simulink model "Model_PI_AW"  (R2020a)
settings: Solver=ode15s  StartTime=0.0  StopTime=tsim  MaxStep=0.1  RelTol=1e-5
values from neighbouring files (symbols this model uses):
  C = Fc*cpc/(Fh*cph)    [calcblock.m]    (also in calcblock2.m; calcblock3.m; eNTU.m = m.c*cp.c/(m.h*cp.h); Main.m = [zeros(1,2*N-1),1])
  d_tstep = 300    [Main.m]    (also in Main_OL.m = 3000; runTestCalcBlk.m; runTransf.m = [500; 50000; 70000; 130000; 50000; 50000]; runTransfOL.m = [500 5000 7000 13000])
  dFh = 0;0.2*Fh    [Main.m]    (also in runTransf.m = 2; runTransfOL.m = 0)
  dTcin = 2    [Main.m]    (also in runTransf.m = 0; runTransfOL.m = 0)
  dThin = 0;2    [Main.m]    (also in runTransf.m = 0; runTransfOL.m = 0)
  Fc0 = 5    [Main.m]    (also in Main_OL.m; runTestCalcBlk.m; runTransf.m; runTransfOL.m)
  Fh = d(1)    [calcblock.m]    (also in calcblock2.m; calcblock3.m; HEXode.m; Main.m = 3)
  Kc = 1/k*tau/(tauC+theta)    (= -0.124875124875)    [Main.m]    (also in runTransf.m = 1/kM(i)*tau(i)/(tauCM(i)+theta(i)); runTransfOL.m = 1/kM(i)*tau(i)/(tauCM(i)+theta(i)))
  nd = size(d0,2)    [Main.m]    (also in Main_OL.m; runTestCalcBlk.m; runTransf.m = size(d0,1); runTransfOL.m)
  np = size(p,2)    [Main.m]    (also in Main_OL.m; runTestCalcBlk.m; runH2Psim.m = length(param); runTransf.m)
  nu = 1    [Main.m]    (also in Main_OL.m; runTestCalcBlk.m; runH2Psim.m = length(u0); runTransf.m)
  nx = size(x0,1)    [Main.m]    (also in Main_OL.m; runTestCalcBlk.m; H2P_Turbine_driven.m = param(end); runTD.m = length(x0))
  p = [N, Fc0, rhoc, rhoh,U,A,cpc,cph]    [Main.m]    (also in Main_OL.m; runTestCalcBlk.m; NonlinearMap.m = [U;A;Fc(i);Fh;cpc;cph;Tcin;Thin]; runTransf.m = [N, Fc0, rhoc, rhoh, U0, A,cpc,cph])
  tauI = min(tau,4*(tauC+theta))    [Main.m]    (also in runTransf.m = min(tau(i), 4*(tauCM(i)+theta(i))); runTransfOL.m = min(tau(i), 4*(tauCM(i)+theta(i))))
  Tcin = d(2)    [calcblock.m]    (also in calcblock2.m; calcblock3.m; HEXode.m; Main.m = 293.15)
  Thin = d(3)    [calcblock.m]    (also in calcblock2.m; calcblock3.m; HEXode.m; Main.m = 343.15)
  Thsp = Thsp0+dThsp    [Main.m]    (also in Main_OL.m = sp(j); runTestCalcBlk.m; runTransf.m = Thsp0; runTransfOL.m = Thsp0)
  Thsp0 = Thend(end)    [Main.m]    (also in Main_OL.m; runTestCalcBlk.m; runTransf.m = x0(end-1);  2.971202611676064e+02; runTransfOL.m = x0(end);  2.971202611676064e+02)
  tstep = 100    [Main.m]    (also in Main_OL.m = 500; runTransf.m = 10000; runTransfOL.m)
  x0 = [Tcend(1:N)'; Thend(1:N)']    [Main.m]    (also in Main_OL.m; runTestCalcBlk.m; runTD.m = [TE0;TD0;TSh0;MD0; MSh0;w0;TA0;0;0;0;0;0;0;0;0;0]; runBD.m = [TE0;TD0;TSh0;MD0; MSh0;w0;TA0;0;0;0;0;0;0;0;0;0])
undefined symbols (not defined in the file or in its folder): HEXode

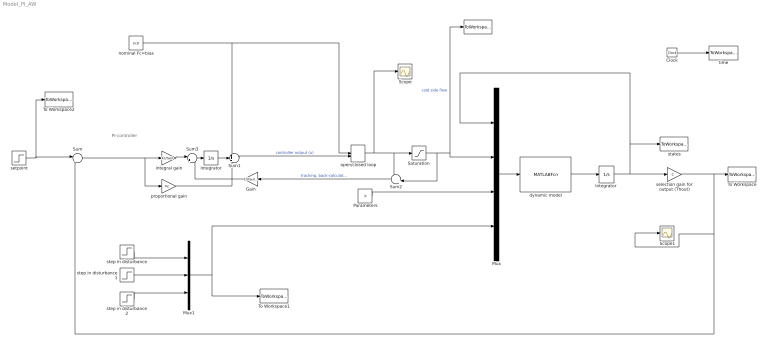
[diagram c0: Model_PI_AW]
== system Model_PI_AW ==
  note: PI-controller
  " " : ToWorkspace  VariableName=uc  SampleTime=-1
  Clock : Clock
  Gain : Gain  Gain=1/(tauI/1)  Multiplication=Matrix(K*u)
  Integrator : Integrator
  "Integrator " : Integrator  InitialCondition=x0
  Mux : Mux
  Mux1 : Mux  Inputs=3
  Parameters : Constant  Value=p
  "Saturation " : Saturate  UpperLimit=inf  LowerLimit=0
  Scope : Scope
  Scope1 : Scope
  Sum : Sum  Inputs=|+-
  Sum1 : Sum  Inputs=+++
  Sum2 : Sum  Inputs=-+|
  Sum3 : Sum  Inputs=|++
  To Workspace : ToWorkspace  VariableName=Thout  SampleTime=-1
  To Workspace1 : ToWorkspace  VariableName=dsim  SampleTime=-1
  To Workspace2 : ToWorkspace  VariableName=Tsp  SampleTime=-1
  dynamic model : MATLABFcn  MATLABFcn=HEXode(u(1:nx),u(nx+1:nx+nu),u(nx+nu+1:nx+nu+np),u(nx+nu+np+1:nx+nu+np+nd))  OutputDimensions=nx  Output1D=off
  integral gain : Gain  Gain=Kc/tauI  Multiplication=Matrix(K*u)
  nominal Fc=bias : Constant  Value=Fc0
  open/closed loop : ManualSwitch  CurrentSetting=0
  proportional gain : Gain  Gain=Kc  Multiplication=Matrix(K*u)
  selection gain for output (Thout) : Gain  Gain=C  Multiplication=Matrix(K*u)
  setpoint : Step  Time=tstep  Before=Thsp0  After=Thsp  SampleTime=0
  states : ToWorkspace  VariableName=T  SampleTime=-1
  step in disturbance : Step  Time=d_tstep(1)  Before=Fh  After=Fh+dFh  SampleTime=0
  step in disturbance1 : Step  Time=d_tstep(2)  Before=Tcin  After=Tcin+dTcin  SampleTime=0
  step in disturbance2 : Step  Time=d_tstep(3)  Before=Thin  After=Thin+dThin  SampleTime=0
  time : ToWorkspace  VariableName=t  SampleTime=-1
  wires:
  dynamic model/1 -> "Integrator "/1
  "Integrator "/1 -> selection gain for output (Thout)/1, states/1, Mux/1
  Mux/1 -> dynamic model/1
  Clock/1 -> time/1
  Parameters/1 -> Mux/3
  Mux1/1 -> Mux/4, To Workspace1/1
  "Saturation "/1 -> Sum2/2, Mux/2, " "/1  "cold side flow"
  Sum/1 -> proportional gain/1, integral gain/1
  integral gain/1 -> Sum3/1
  Integrator/1 -> Sum1/2
  selection gain for output (Thout)/1 -> Scope1/1, Sum/2, To Workspace/1
  open/closed loop/1 -> Scope/1, "Saturation "/1, Sum2/1
  nominal Fc=bias/1 -> open/closed loop/1, Sum1/1
  proportional gain/1 -> Sum1/3
  Sum1/1 -> open/closed loop/2  "controller output (u)"
  setpoint/1 -> To Workspace2/1, Sum/1
  Sum3/1 -> Integrator/1
  Sum2/1 -> Gain/1  "tracking. back-calculation"
  Gain/1 -> Sum3/2
  step in disturbance2/1 -> Mux1/3
  step in disturbance1/1 -> Mux1/2
  step in disturbance/1 -> Mux1/1
